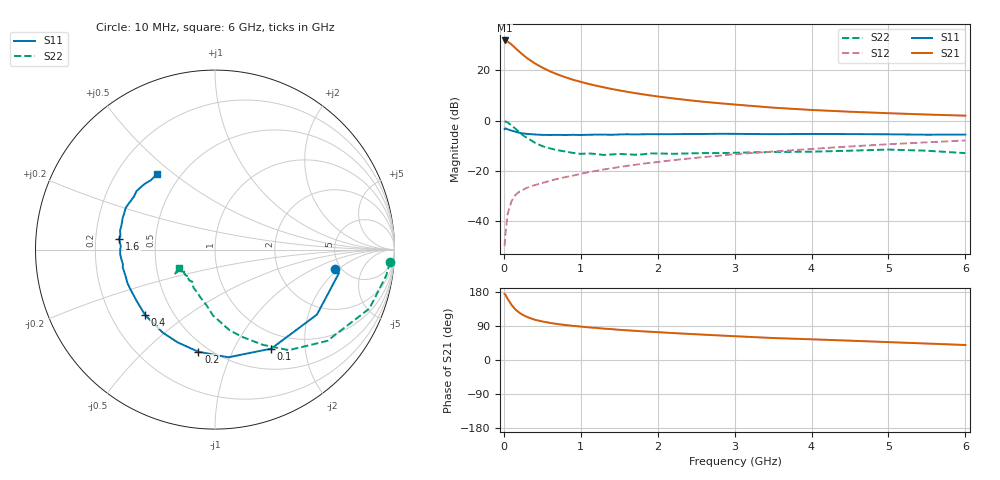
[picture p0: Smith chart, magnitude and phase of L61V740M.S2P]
!  INFINEON TECHNOLOGIES Small Signal Semiconductors
! BFR380L3 , Si-NPN RF-Transistor in TSLP-3-1
!  Vce=1.75 V,  Ic=40 mA
! Common Emitter S-Parameters:  07. March 2005
#  GHz  S  MA  R  50
! f  S11  S21  S12  S22
! GHz  Mag  Ang  Mag  Ang  Mag  Ang  Mag  Ang
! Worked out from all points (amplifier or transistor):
!   36 points, 10 MHz to 6 GHz, reference 50 ohm
!   highest |S21| = 31.9 dB at 10 MHz (marker M1)
!   |S21| within 3 dB of that: start of sweep to 149.5 MHz
!   unconditionally stable (mu >= 1): 1.641 GHz to 4.898 GHz
!   at 250 MHz: K = 0.44, MSG = 26.8 dB, |S12| = -27.5 dB
!   at 1.4 GHz: K = 0.98, MSG = 15.8 dB, |S12| = -18.9 dB
!   at 6 GHz: K = 0.98, MSG = 4.9 dB, |S12| = -7.9 dB
!   S11 on the Smith chart (normalised r, x): 10 MHz: 4.47, -1.83; 100 MHz: 0.77, -1.42; 200 MHz: 0.44, -0.75; 400 MHz: 0.35, -0.35; 1.6 GHz: 0.30, +0.05; 6 GHz: 0.37, +0.44
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0.01  0.6802 -9.3  39.38 174.4  0.0032 83.7  0.9772 -4.1
0.02  0.7027 -10.8  39.25 172.5  0.0054 85.2  0.965 -8.6
0.05  0.6736 -32.5  37.36 161.1  0.0142 76.3  0.9209 -20.9
0.1  0.6346 -60.4  32.73 145.5  0.0252 65.8  0.8063 -39.1
0.15  0.6047 -82.9  27.83 133.5  0.0333 57.6  0.6952 -53.7
0.2  0.5768 -99.2  23.61 124.9  0.0386 55.5  0.5949 -63.2
0.25  0.5572 -112.0  20.32 118.7  0.0424 52.5  0.5094 -72.7
0.3  0.5464 -122.1  17.6 113.6  0.0463 51.7  0.4569 -79.7
0.4  0.5333 -137.0  13.86 106.4  0.0521 52.3  0.3671 -91.8
0.5  0.5218 -146.8  11.38 101.7  0.0578 53.3  0.3121 -98.9
0.6  0.5205 -154.1  9.566 97.9  0.0637 54.5  0.2815 -106.1
0.7  0.5222 -159.1  8.299 94.9  0.0699 56.3  0.2579 -112.9
0.9  0.5236 -168.9  6.514 90.1  0.0809 59.4  0.2285 -123.9
1.1  0.5251 -174.6  5.392 86.2  0.0946 61.3  0.2235 -129.4
1.3  0.5284 179.8  4.603 82.8  0.1075 62.3  0.2084 -137.2
1.6  0.5371 173.4  3.759 78.3  0.1263 63.0  0.2153 -143.7
2.2  0.5396 163.9  2.777 71.1  0.1641 64.2  0.2194 -146.1
2.8  0.5488 155.4  2.226 64.8  0.2014 64.2  0.227 -151.6
3.5  0.5397 146.9  1.817 58.0  0.2438 62.2  0.2387 -150.3
4.5  0.5416 140.8  1.507 51.0  0.3075 60.4  0.2533 -149.4
5.5  0.5266 132.7  1.326 43.4  0.3718 56.5  0.2528 -149.3
6  0.5302 127.5  1.259 39.6  0.4039 54.3  0.2265 -152.6
